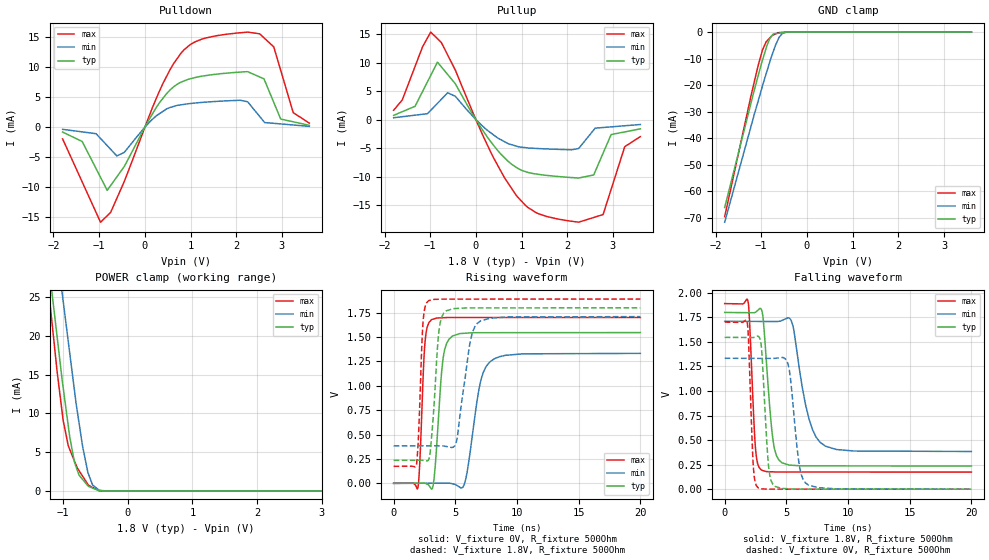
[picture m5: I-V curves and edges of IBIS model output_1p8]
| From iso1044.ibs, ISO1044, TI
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|   output_1p8 Model
[Model]   output_1p8
Model_type   3-state
Polarity   Inverting
Vmeas = 0.9
Vref = 0
Cref = 2pF
Rref = 100000
|   typ   min   max
C_comp   1.293pF   1.246pF   1.386pF
|C_comp_pullup   1.275pF   1.258pF   1.323pF
|C_comp_pulldown   1.218pF   1.207pF   1.275pF
|  Where Nom  PVT is Nominal Process, 1.8V,  27C
|   Fast PVT is Strong Process,  1.89, -40C
|   Slow PVT is Weak Process,   1.71V, 150C
[Voltage Range]   1.8   1.71   1.89
|Junction Temperature
[Temperature Range]   27   150   -40
[Pullup Reference]   1.8   1.71   1.89
[Pulldown Reference]   -0   0   -0
[Power Clamp Reference]   1.8   1.71   1.89
[GND Clamp Reference]   0   0   0
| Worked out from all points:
|   slope of the pulldown table from 0 to 0.27 V, typ, clamps not added: 76.8 ohm
|   slope of the pullup table from 0 to 0.27 V, typ, clamps not added: 82.6 ohm
|   GND clamp passes 1 mA (typ) near -0.75 V on its own axis
|   POWER clamp passes 1 mA (typ) near -0.65 V on its own axis
|   falling waveform, V_fixture 1.8V, R_fixture 500Ohm: 20-80 % time 594ps typ, 1.2ns min, 367ps max; typ from 1.8 V to 0.236 V
|   rising waveform, V_fixture 0V, R_fixture 500Ohm: 20-80 % time 519ps typ, 948ps min, 328ps max; typ from 0 V to 1.55 V
|   rising waveform, V_fixture 1.8V, R_fixture 500Ohm: 20-80 % time 487ps typ, 868ps min, 305ps max; typ from 0.236 V to 1.8 V
|   falling waveform, V_fixture 0V, R_fixture 500Ohm: 20-80 % time 419ps typ, 641ps min, 297ps max; typ from 1.55 V to 0 V
[Pulldown]
|   Voltage   I(typ)   I(min)   I(max)
-1.8V     -806.3uA   -351.8uA   -1.947mA
-1.372V   -2.375mA   -775uA     -9.106mA
-970.1mV  -8.348mA   -1.871mA   -15.83mA
-823.7mV  -10.52mA   -3.067mA   -14.75mA
-613.1mV  -8.28mA    -4.788mA   -11.85mA
321.3mV   4.097mA    2.26mA     6.051mA
790.6mV   7.512mA    3.734mA    12.34mA
2.25V     9.259mA    4.238mA    15.86mA
2.607V    8.063mA    920.7uA    14.91mA
2.822V    4.144mA    648.9uA    13.39mA
3.248V    904.8uA    372.6uA    2.426mA
3.6V      315.5uA    144.1uA    678uA
[GND Clamp]
|   Voltage   I(typ)   I(min)   I(max)
-1.8V     -66.17mA   -71.69mA   -69.59mA
-1.222V   -26.61mA   -35.44mA   -23.87mA
-1.071V   -16.68mA   -26.16mA   -12.77mA
-972.9mV  -10.58mA   -20.31mA   -6.741mA
-892mV    -6.036mA   -15.67mA   -3.651mA
-802.3mV  -2.066mA   -10.64mA   -2.027mA
-766.2mV  -1.327mA   -8.794mA   -1.375mA
-687.9mV  -577.7uA   -4.937mA   -700.9uA
-607.9mV  -384.2uA   -1.942mA   -204.8uA
-539.2mV  -218uA     -539.4uA   -117uA
-449.9mV  -2.005uA   -59.78uA   -2.825uA
3.6V      0A         0A         0A
[Pullup]
|   Voltage   I(typ)   I(min)   I(max)
-1.8V     749.2uA    331.9uA    1.645mA
-1.332V   2.34mA     778.9uA    9.319mA
-988.5mV  7.758mA    1.633mA    15.35mA
-841.3mV  10.08mA    2.854mA    14.19mA
-617.7mV  7.912mA    4.71mA     11.33mA
861.2mV   -8.24mA    -4.59mA    -13.03mA
2.25V     -10.24mA   -5.059mA   -17.98mA
2.579V    -9.7mA     -1.81mA    -17.15mA
2.784V    -5.874mA   -1.382mA   -16.64mA
2.96V     -2.616mA   -1.268mA   -12.24mA
3.258V    -2.15mA    -1.074mA   -4.738mA
3.6V      -1.617mA   -852.7uA   -2.974mA
[POWER Clamp]
|   Voltage   I(typ)   I(min)   I(max)
-1.8V     73.64mA    80.72mA    75.63mA
-1.242V   30.77mA    40.89mA    27.23mA
-1.188V   26.64mA    37.05mA    22.93mA
-1.162V   24.73mA    35.15mA    20.8mA
-1.015V   14.25mA    25.48mA    10.09mA
-920.6mV  8.33mA     19.22mA    5.79mA
-828mV    3.775mA    13.11mA    3.905mA
-698.9mV  1.476mA    5.701mA    1.892mA
-610.3mV  590.3uA    2.206mA    755.6uA
-546mV    369.9uA    774.3uA    454uA
-355.8mV  4.932uA    20.1uA     2.334uA
3.6V      0A         0A         0A
[Ramp]
R_load = 500
|   typ   min   max
dV/dt_r   0.927695/5.15062e-10   0.799772/9.45208e-10   1.02082/3.27709e-10
dV/dt_f   0.938426/5.92453e-10   0.795755/1.19026e-09   1.0295/3.6509e-10
[Falling Waveform]
V_fixture = 1.8V
V_fixture_min = 1.71V
V_fixture_max = 1.89V
R_fixture = 500Ohm
C_fixture = 0F
|   Time   V(typ)   V(min)   V(max)
0s        1.8V       1.71V      1.89V
1.881ns   1.798V     1.709V     1.918V
2.491ns   1.802V     1.709V     425.2mV
2.971ns   1.83V      1.708V     194.9mV
3.907ns   510mV      1.708V     176.3mV
4.637ns   269.7mV    1.718V     174.6mV
5.419ns   243.8mV    1.709V     174.6mV
6.826ns   237mV      718.8mV    174.6mV
8.156ns   236.9mV    438.9mV    174.5mV
20ns      236mV      383.7mV    174.2mV
[Rising Waveform]
V_fixture = 0V
V_fixture_min = 0V
V_fixture_max = 0V
R_fixture = 500Ohm
C_fixture = 0F
|   Time   V(typ)   V(min)   V(max)
0s        -701.1nV   1.066uV    -3.78nV
1.962ns   1.104mV    579.3uV    -49.18mV
2.531ns   1.424mV    747.1uV    1.431V
3.061ns   -59.26mV   903.4uV    1.678V
4.007ns   1.28V      1.182mV    1.699V
4.767ns   1.51V      -4.802mV   1.701V
5.729ns   1.539V     -9.799mV   1.701V
7.066ns   1.545V     1.056V     1.701V
8.166ns   1.545V     1.278V     1.701V
20ns      1.546V     1.333V     1.701V
[Rising Waveform]
V_fixture = 1.8V
V_fixture_min = 1.71V
V_fixture_max = 1.89V
R_fixture = 500Ohm
C_fixture = 0F
|   Time   V(typ)   V(min)   V(max)
0s        236mV      383.7mV    174.2mV
1.846ns   237.1mV    384.3mV    192.2mV
2.381ns   235.7mV    384.4mV    1.652V
2.821ns   241mV      384.6mV    1.872V
3.677ns   1.569V     384.8mV    1.888V
4.267ns   1.769V     377.9mV    1.89V
5.071ns   1.793V     420.3mV    1.89V
6.237ns   1.799V     1.472V     1.89V
7.046ns   1.799V     1.666V     1.89V
20ns      1.8V       1.71V      1.89V
[Falling Waveform]
|Gnd
V_fixture = 0V
V_fixture_min = 0V
V_fixture_max = 0V
R_fixture = 500Ohm
C_fixture = 0F
|   Time   V(typ)   V(min)   V(max)
0s        1.546V     1.333V     1.701V
1.826ns   1.545V     1.332V     1.695V
2.321ns   1.544V     1.332V     231.8mV
2.711ns   1.558V     1.332V     14.28mV
3.577ns   211.6mV    1.332V     392.6uV
4.097ns   27.56mV    1.333V     227.1uV
5.179ns   3.966mV    1.252V     211.6uV
6.077ns   855.8uV    222.7mV    198.8uV
6.786ns   812.1uV    41.64mV    188.7uV
20ns      -138nV     980.3nV    -4.639nV
